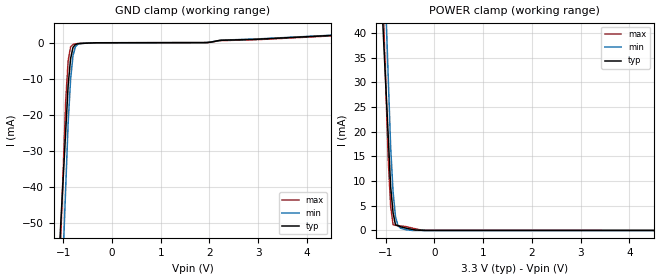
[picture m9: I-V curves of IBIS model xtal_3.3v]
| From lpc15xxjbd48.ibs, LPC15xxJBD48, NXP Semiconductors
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[Model] xtal_3.3v
Model_type Input
Vinl = 990.000mV
Vinh = 2.31000V
C_comp 2.00000pF 2.00000pF 2.00000pF
| variable typ   min   max
[Voltage Range] 3.30000V 3.00000V 3.60000V
[POWER Clamp Reference] 3.30000V 3.00000V 3.60000V
[GND Clamp Reference] 0.00000V 0.00000V 0.00000V
[Temperature Range]   25   85   -40
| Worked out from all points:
|   GND clamp passes 1 mA (typ) near -0.78 V on its own axis
|   POWER clamp passes 1 mA (typ) near -0.75 V on its own axis
[GND Clamp]
-3.3V     -620.4mA   -882.1mA   -889.8mA
-950mV    -24.52mA   -40.16mA   -16.13mA
-900mV    -11.84mA   -22.25mA   -4.99mA
-850mV    -4.427mA   -10.2mA    -1.199mA
-800mV    -1.281mA   -3.529mA   -459.8uA
-750mV    -464.4uA   -1.068mA   -339.6uA
-700mV    -268.4uA   -417.5uA   -219.4uA
-500mV    -107uA     -62.19uA   -100.9uA
1.9V      45.69uA    21.6uA     25.11uA
2.25V     684uA      732.8uA    595.8uA
3V        983.4uA    1.069mA    867.8uA
6.6V      3.468mA    3.504mA    3.342mA
[POWER Clamp]
-3.3V     503.3mA    701.1mA    719.8mA
-1.15V    60.35mA    88.16mA    74.48mA
-1.05V    39.75mA    59.65mA    44.46mA
-950mV    19.15mA    31.14mA    14.45mA
-900mV    8.845mA    16.89mA    4.93mA
-850mV    3.57mA     7.735mA    1.178mA
-800mV    1.116mA    2.763mA    1.054mA
-750mV    1.001mA    983.6uA    929.2uA
-700mV    756.5uA    489.4uA    929.2uA
-450mV    201.9uA    55.78pA    471.8uA
-150mV    0A         0A         64.42uA
6.6V      0A         0A         0A
